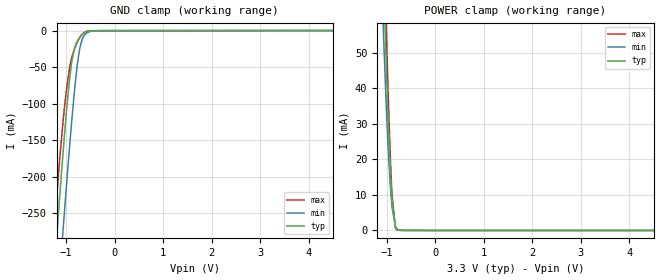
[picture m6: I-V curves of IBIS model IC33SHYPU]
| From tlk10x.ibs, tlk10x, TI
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|   Model
[Model]   IC33SHYPU
Model_type   Input
Vinl = 0.99
Vinh = 2.31
|   typ   min   max
C_comp   1.475pF   1.444pF   1.523pF
[Voltage Range]   3.3   3   3.6
[Temperature Range]   25   125   -40
[Power Clamp Reference]   3.3   3   3.6
[GND Clamp Reference]   -0   -0   -0
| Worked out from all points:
|   GND clamp passes 1 mA (typ) near -0.55 V on its own axis
|   POWER clamp passes 1 mA (typ) near -0.82 V on its own axis
[GND Clamp]
|   Voltage   I(typ)   I(min)   I(max)
-3.3V     -2.326A    -2.431A    -2.267A
-1.251V   -331.2mA   -441.1mA   -274.2mA
-1.142V   -233mA     -341.3mA   -181.8mA
-1.063V   -164.8mA   -270.5mA   -122.4mA
-983.4mV  -102mA     -201.9mA   -74.73mA
-884.4mV  -41.86mA   -121.8mA   -36.29mA
-825mV    -23.23mA   -79.08mA   -23.97mA
-745.8mV  -11.77mA   -34.45mA   -12.26mA
-686.4mV  -6.561mA   -15.09mA   -6.001mA
-607.2mV  -2.362mA   -4.949mA   -1.611mA
-270.6mV  -100.6uA   -77.26uA   -153.5uA
6.59V     0A         0A         0A
[POWER Clamp]
|   Voltage   I(typ)   I(min)   I(max)
-3.3V     1.527A     1.443A     1.596A
-1.082V   79.33mA    60.58mA    96.2mA
-1.063V   69.44mA    52.81mA    84.78mA
-1.053V   64.66mA    49.08mA    79.19mA
-1.013V   46.79mA    35.24mA    57.85mA
-1.003V   42.67mA    32.07mA    52.82mA
-973.5mV  31.2mA     23.28mA    38.7mA
-933.9mV  18.23mA    13.56mA    22.51mA
-894.3mV  8.509mA    6.639mA    10.13mA
-825mV    1.056mA    1.236mA    823.2uA
-785.4mV  257.7uA    415.7uA    152uA
6.59V     0A         0A         0A
